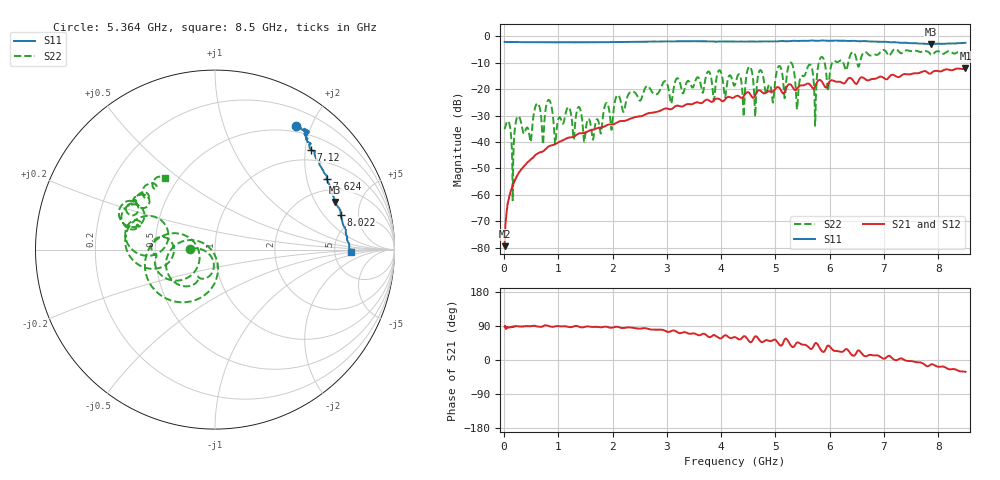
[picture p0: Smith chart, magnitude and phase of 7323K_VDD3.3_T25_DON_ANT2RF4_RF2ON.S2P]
!Agilent Technologies,E5071C,MY46417908,A.11.23
!Date: Mon Jan 18 17:06:26 2021
!Data & Calibration Information:
!Freq	S11:SOLT2(ON)	S21:SOLT2(ON)	S12:SOLT2(ON)	S22:SOLT2(ON)
!PortZ  Port1:50+j0  Port2:50+j0
!Above PortZ is port z conversion or system Z0 setting when saving the data.
!When reading, reference impedance value at option line is always used.
# Hz S dB R 50
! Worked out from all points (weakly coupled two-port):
!   1601 points, 10 MHz to 8.5 GHz, reference 50 ohm
!   highest |S21| = -12.06 dB at 8.5 GHz (marker M1); lowest = -79.5 dB at 10 MHz (marker M2)
!   lowest |S11| = -2.8 dB at 7.869 GHz (marker M3), VSWR 6.16, Z = 134 + j148 ohm
!   |S11| at or under -10 dB: nowhere
!   |S22| runs from -62.1 to -4.8 dB; largest |S21 - S12| = 0.0035
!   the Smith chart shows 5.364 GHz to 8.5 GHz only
!   S11 on the Smith chart (normalised r, x): 5.364 GHz: 0.41, +1.78; 7.12 GHz: 0.76, +2.11; 7.624 GHz: 1.54, +2.65; 8.022 GHz: 3.73, +3.04; 8.5 GHz: 7.28, -0.49
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1e7  -2.04 179.7  -79.47 87.8  -79.83 81.3  -35.13 6.0
1.58575e8  -2.10 176.0  -56.59 86.7  -56.49 87.7  -62.10 -142.1
3.124562e8  -2.16 172.3  -50.47 88.2  -50.51 88.1  -32.49 -14.7
4.822562e8  -2.17 168.2  -46.81 89.2  -46.81 89.1  -39.51 5.8
6.149125e8  -2.18 164.9  -44.44 88.4  -44.42 88.4  -25.30 -10.8
7.210375e8  -2.18 162.4  -43.49 89.2  -43.50 89.4  -40.40 149.9
8.218562e8  -2.21 159.8  -41.67 89.9  -41.65 90.0  -24.02 -1.4
9.492062e8  -2.21 156.4  -40.73 88.9  -40.75 89.2  -40.02 -12.8
1.426769e9  -2.20 143.9  -36.64 86.1  -36.65 85.9  -29.84 -70.5
2.843538e9  -1.94 111.1  -28.39 80.1  -28.39 80.1  -21.40 -17.3
4.255e9  -1.93 84.9  -22.84 60.3  -22.85 60.2  -18.29 -121.5
4.944812e9  -1.85 65.2  -20.93 51.7  -20.92 51.6  -23.98 -125.2
5.279106e9  -1.73 56.7  -18.23 39.0  -18.20 39.1  -9.88 -116.2
5.364006e9  -1.67 56.8  -20.34 40.0  -20.33 39.8  -17.01 178.7
5.671769e9  -1.53 53.2  -19.20 29.8  -19.15 29.8  -11.92 -177.4
5.730138e9  -1.61 53.4  -19.03 43.7  -19.01 43.6  -33.82 -177.2
7.088538e9  -2.17 47.6  -15.55 11.1  -15.61 11.0  -7.28 155.8
7.120375e9  -2.24 46.2  -14.78 9.1  -14.80 9.0  -6.79 163.8
7.624469e9  -2.65 32.3  -13.92 -6.0  -13.93 -5.9  -5.58 148.7
7.868556e9  -2.85 21.6  -13.91 -11.7  -13.95 -11.5  -6.96 144.6
8.022438e9  -2.77 15.4  -13.19 -18.2  -13.23 -18.2  -5.76 141.8
8.5e9  -2.39 -1.1  -12.06 -31.0  -12.15 -31.1  -6.25 124.8
